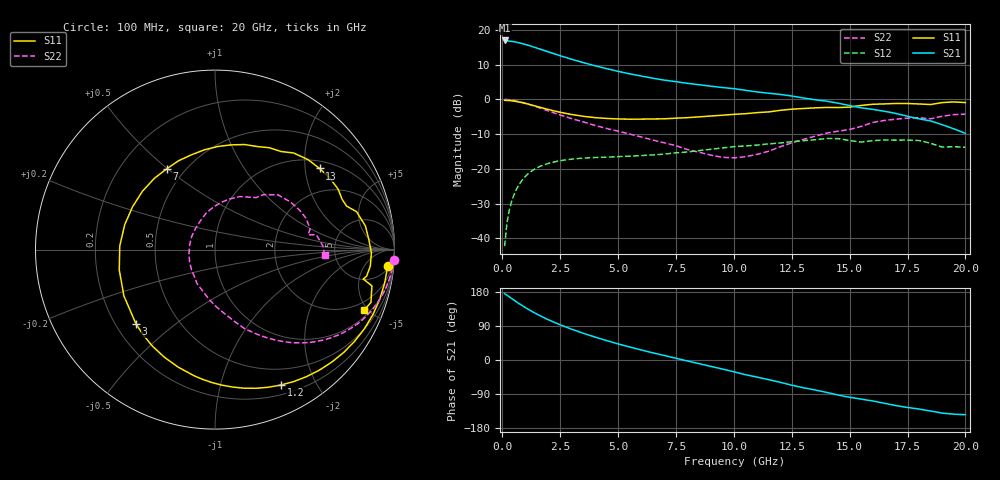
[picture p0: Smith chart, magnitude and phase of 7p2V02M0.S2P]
! Infineon Technologies  Discrete & RF Semiconductors
! bfp620
! VCE =  2.0 V,  IC =  2.0 mA
! Common Emitter S-Parameters:  Sep 2002
# GHz  S  MA  R  50
!  f  S11  S21  S12  S22
! GHz  MAG  ANG  MAG  ANG  MAG  ANG  MAG  ANG
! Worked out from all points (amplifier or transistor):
!   59 points, 100 MHz to 20 GHz, reference 50 ohm
!   highest |S21| = 16.9 dB at 100 MHz (marker M1)
!   |S21| within 3 dB of that: start of sweep to 1.862 GHz
!   unconditionally stable (mu >= 1): 5.765 GHz to 15.66 GHz; 17.6 GHz to end of sweep
!   at 1 GHz: K = 0.16, MSG = 19.0 dB, |S12| = -22.2 dB
!   at 5.5 GHz: K = 0.97, MSG = 11.8 dB, |S12| = -16.4 dB
!   at 20 GHz: K = 1.34, MAG = -1.5 dB, |S12| = -13.8 dB
!   S11 on the Smith chart (normalised r, x): 100 MHz: 7, -18; 1.2 GHz: 0.31, -1.56; 3 GHz: 0.28, -0.37; 7 GHz: 0.40, +0.50; 13 GHz: 1.21, +2.39; 20 GHz: 1.37, -4.76
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0.1  0.9665 -5.5  7.034 175.1  0.0077 84.5  0.9975 -3.3
0.3  0.9586 -16.8  6.887 166.7  0.0252 80.3  0.9853 -9.6
0.5  0.9421 -27.9  6.734 158.1  0.0419 74.2  0.9638 -15.8
0.7  0.9178 -38.7  6.538 149.8  0.0575 67.7  0.934 -21.7
0.9  0.8883 -49.1  6.294 142.0  0.0714 61.4  0.8978 -27.2
1.2  0.8393 -64.0  5.878 131.0  0.0893 52.7  0.8368 -34.6
1.6  0.7728 -82.5  5.322 117.8  0.1072 42.8  0.7542 -43.0
2  0.7121 -99.5  4.807 106.0  0.1198 34.6  0.6787 -49.9
2.4  0.6626 -115.2  4.344 95.4  0.1289 27.8  0.6117 -55.8
3  0.6044 -136.7  3.765 81.2  0.1377 19.5  0.5279 -63.5
3.5  0.5695 -153.0  3.377 70.5  0.1428 13.8  0.473 -69.2
4  0.5454 -168.0  3.042 60.6  0.1453 8.9  0.4207 -74.2
5  0.5218 164.6  2.529 42.5  0.1497 2.2  0.3478 -83.5
6  0.5188 141.2  2.163 26.5  0.155 -2.8  0.2873 -94.9
7  0.5243 120.9  1.889 11.9  0.1629 -6.6  0.2365 -107.9
9  0.575 88.3  1.546 -16.8  0.1909 -16.5  0.1573 -154.4
10.5  0.6207 67.7  1.348 -38.7  0.2132 -27.5  0.1494 150.1
13  0.7373 37.8  1.046 -73.2  0.2537 -46.2  0.2647 82.7
13.5  0.7534 32.1  0.986 -79.0  0.2621 -50.9  0.2939 73.8
15  0.7721 18.3  0.814 -98.4  0.255 -70.3  0.3686 51.8
17  0.8716 -1.2  0.626 -120.2  0.2586 -82.9  0.5179 25.6
20  0.8979 -22.0  0.324 -144.3  0.2044 -104.8  0.612 -2.9
